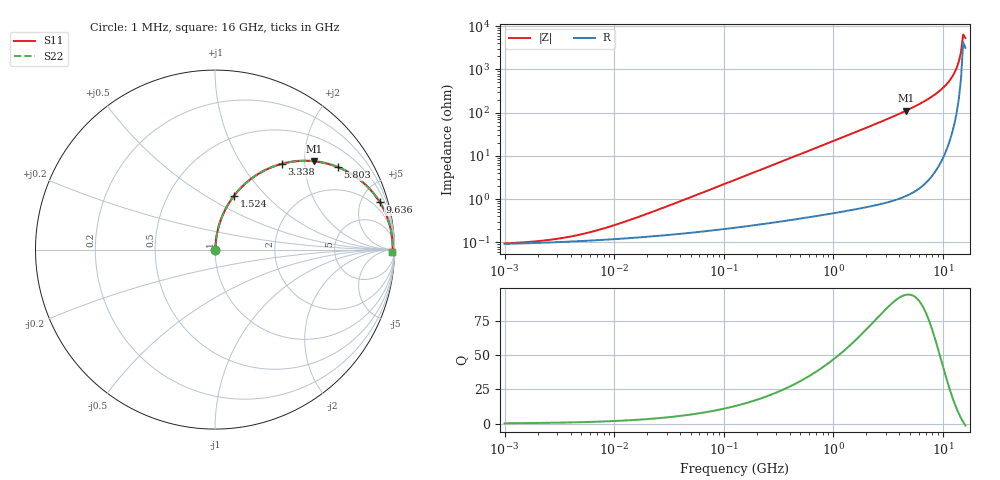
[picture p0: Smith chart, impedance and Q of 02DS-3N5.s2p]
# MHz S MA R 50
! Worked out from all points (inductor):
!   211 points, 1 MHz to 16 GHz, reference 50 ohm
!   read as one part in series: L = 3.5 nH near 18.25 MHz
!   highest Q = 93.8 at 4.609 GHz (marker M1), where L = 3.84 nH
!   self-resonance near 15.28 GHz
!   S11 on the Smith chart (normalised r, x): 1 MHz: 1.00, +0.00; 1.524 GHz: 1.01, +0.68; 3.338 GHz: 1.02, +1.54; 5.803 GHz: 1.03, +2.96; 9.636 GHz: 1.15, +6.86; 16 GHz: open
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1  0.000948 13.4  0.9991 -0.0  0.9991 -0.0  0.000948 13.4
2.51416  0.001137 29.0  0.999 -0.0  0.999 -0.0  0.001137 29.0
5.25662  0.001582 46.8  0.9989 -0.1  0.9989 -0.1  0.001582 46.8
10.4954  0.002598 62.4  0.9988 -0.1  0.9988 -0.1  0.002598 62.4
26.3872  0.005968 75.8  0.9986 -0.3  0.9986 -0.3  0.005968 75.8
132.458  0.02914 84.0  0.9974 -1.7  0.9974 -1.7  0.02914 84.0
333.021  0.07291 83.4  0.9943 -4.2  0.9943 -4.2  0.07291 83.4
664.915  0.1444 80.1  0.9856 -8.3  0.9856 -8.3  0.1444 80.1
1524.47  0.319 70.4  0.9424 -18.6  0.9424 -18.6  0.319 70.4
2204.33  0.441 63.0  0.8914 -26.2  0.8914 -26.2  0.441 63.0
3187.38  0.5872 53.4  0.8026 -36.0  0.8026 -36.0  0.5872 53.4
3337.74  0.6064 52.0  0.7882 -37.3  0.7882 -37.3  0.6064 52.0
4608.83  0.7393 41.7  0.6656 -47.7  0.6656 -47.7  0.7393 41.7
5803.48  0.8247 33.8  0.5566 -55.6  0.5566 -55.6  0.8247 33.8
7652.55  0.9069 24.1  0.409 -65.1  0.409 -65.1  0.9069 24.1
9636.16  0.9545 16.2  0.2783 -72.6  0.2783 -72.6  0.9545 16.2
11065.3  0.9734 11.4  0.1985 -76.6  0.1985 -76.6  0.9734 11.4
12706.4  0.9851 6.8  0.1185 -79.4  0.1185 -79.4  0.9851 6.8
13933.5  0.989 3.7  0.06547 -78.4  0.06547 -78.4  0.989 3.7
14590.9  0.9897 2.2  0.03938 -73.8  0.03938 -73.8  0.9897 2.2
15279.2  0.9897 0.7  0.01546 -47.9  0.01546 -47.9  0.9897 0.7
16000  0.9889 -0.9  0.01859 52.9  0.01859 52.9  0.9889 -0.9
